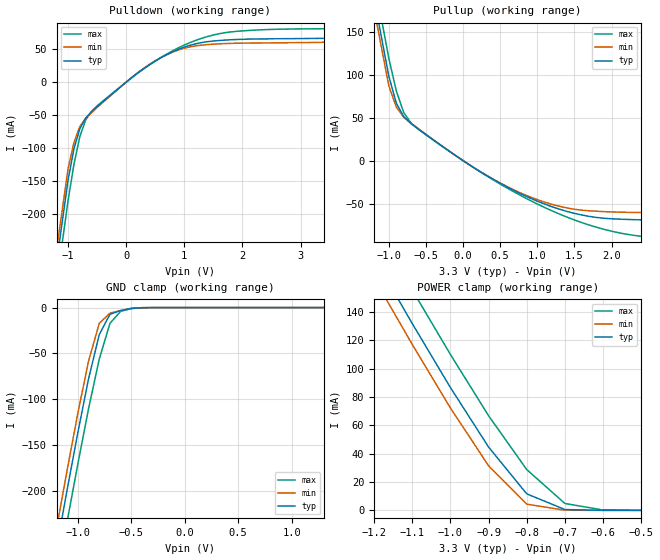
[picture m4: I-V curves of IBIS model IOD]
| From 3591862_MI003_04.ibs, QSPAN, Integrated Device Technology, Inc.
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|   Model IOD
[Model]   IOD
Model_type   I/O
Polarity   Non-Inverting
Vinl =   0.8000V
Vinh =   2.0000V
C_comp   5.00pF   5.00pF   5.00pF
[Voltage Range]   3.3000V   3.0000V   4.0000V
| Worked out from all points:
|   slope of the pulldown table from 0 to 0.495 V, typ, clamps not added: 15.6 ohm
|   slope of the pullup table from 0 to 0.495 V, typ, clamps not added: 19 ohm
|   GND clamp passes 1 mA (typ) near -0.50 V on its own axis
|   POWER clamp passes 1 mA (typ) near -0.70 V on its own axis
[Pulldown]
| voltage   I(typ)   I(min)   I(max)
-3.3V     -1.694A    -1.674A    -1.726A
-1.5V     -464.7mA   -443.3mA   -499.1mA
-1V       -148.3mA   -131mA     -179.4mA
-900mV    -101.4mA   -92mA      -124.9mA
-800mV    -71.35mA   -67.54mA   -83.38mA
-700mV    -54.61mA   -55.52mA   -57.94mA
-300mV    -22.15mA   -23.01mA   -21.41mA
300mV     20.4mA     20.95mA    20.07mA
700mV     41.89mA    41.82mA    42.76mA
1.2V      58.32mA    55.16mA    63.56mA
1.7V      63.86mA    58.59mA    75.13mA
3.4V      66.51mA    60.6mA     81.17mA
[Pullup]
| voltage   I(typ)   I(min)   I(max)
-3.3V     1.219A     1.205A     1.24A
-1.5V     325.7mA    311.2mA    349mA
-1V       97.95mA    86.62mA    118.7mA
-900mV    66.92mA    62.39mA    81.13mA
-800mV    51.19mA    50.49mA    55.92mA
-700mV    42.9mA     43.48mA    43.54mA
-600mV    36.5mA     37.05mA    36.37mA
100mV     -5.631mA   -5.673mA   -5.695mA
700mV     -35.26mA   -34.53mA   -36.94mA
1.2V      -53.58mA   -50.8mA    -58.38mA
1.7V      -64.75mA   -58.26mA   -74.81mA
2.4V      -68.76mA   -60.18mA   -87.86mA
[GND_clamp]
| voltage   I(typ)   I(min)   I(max)
-3.3V     -1.693A    -1.673A    -1.725A
-1.2V     -263.1mA   -241.4mA   -297.9mA
-1.1V     -198.7mA   -177.1mA   -233.4mA
-1V       -136.2mA   -115.1mA   -170.5mA
-900mV    -77.68mA   -58.22mA   -110.3mA
-800mV    -29.37mA   -17.18mA   -56.11mA
-700mV    -7.314mA   -6.096mA   -17.15mA
-600mV    -3.242mA   -3.24mA    -4.049mA
-500mV    -896.8uA   -801.3uA   -1.075mA
-400mV    -106.5uA   -71.5uA    -178.6uA
1.3V      30.52uA    24.92uA    33.55uA
[POWER_clamp]
| voltage   I(typ)   I(min)   I(max)
-3.3V     1.218A     1.204A     1.24A
-1.2V     178.7mA    163.9mA    202.3mA
-1.1V     131.9mA    117.2mA    155.6mA
-1V       86.74mA    72.3mA     110.1mA
-900mV    44.73mA    31.52mA    66.84mA
-800mV    11.68mA    4.404mA    28.8mA
-700mV    608.8uA    114.5uA    4.876mA
-600mV    47.41uA    24.43uA    269uA
-500mV    34.93uA    23.13uA    49.9uA
[Ramp]
| variable   typ   min   max
dV/dt_r   1.3908/0.4611n   1.2594/0.4638n   1.7040/0.4368n
dV/dt_f   1.4599/0.3721n   1.3370/0.3359n   1.7622/0.3609n
R_load = 50.0000
| End [Model] IOD
